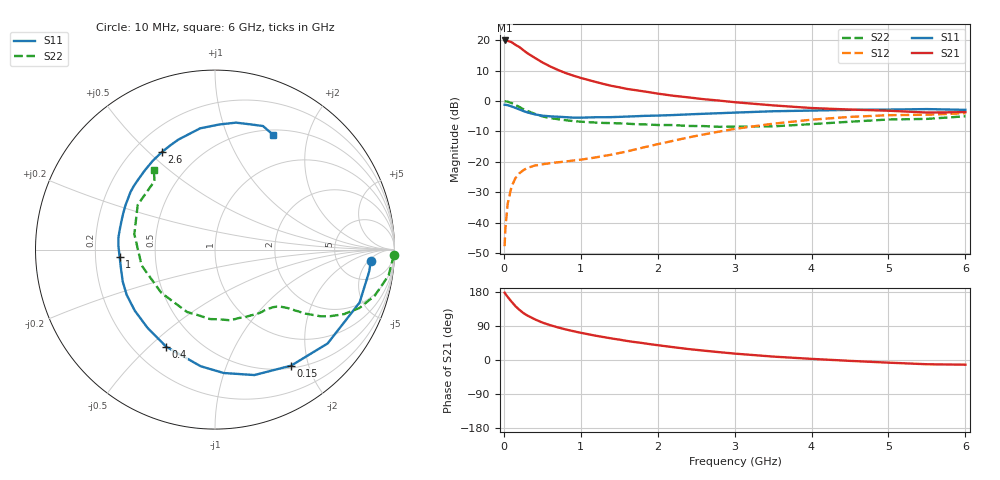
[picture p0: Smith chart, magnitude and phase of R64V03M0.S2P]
! SIEMENS Small Signal Semiconductors
! BFR193
! Si NPN RF Bipolar Junction Transistor in SOT23
! VCE = 4 V  IC = 3 mA
! Common Emitter S-Parameters:  May  1996
# GHz  S  MA  R  50
!  f  S11  S21  S12  S22
! GHz  MAG  ANG  MAG  ANG  MAG  ANG  MAG  ANG
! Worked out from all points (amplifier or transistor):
!   36 points, 10 MHz to 6 GHz, reference 50 ohm
!   highest |S21| = 20.0 dB at 10 MHz (marker M1)
!   |S21| within 3 dB of that: start of sweep to 244.1 MHz
!   unconditionally stable (mu >= 1): 1.043 GHz to 2.02 GHz
!   at 250 MHz: K = 0.31, MSG = 19.8 dB, |S12| = -22.8 dB
!   at 1.4 GHz: K = 1.10, MAG = 9.4 dB, |S12| = -17.6 dB
!   at 6 GHz: K = 0.98, MSG = 0.2 dB, |S12| = -4.0 dB
!   S11 on the Smith chart (normalised r, x): 10 MHz: 11, -6; 150 MHz: 0.54, -1.73; 400 MHz: 0.33, -0.57; 1 GHz: 0.31, -0.03; 2.6 GHz: 0.31, +0.55; 6 GHz: 0.56, +1.47
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0.01  0.8696 -4.2  9.946 177.6  0.0041 87.6  0.9953 -1.7
0.02  0.8681 -7.9  9.763 174.5  0.0081 83.7  0.9914 -3.3
0.05  0.858 -20.1  9.777 166.5  0.0205 79.3  0.9781 -8.4
0.1  0.8169 -39.8  9.339 153.9  0.0391 69.2  0.927 -16.0
0.15  0.7733 -56.7  8.433 142.2  0.0538 61.4  0.8684 -22.0
0.2  0.7325 -72.6  7.772 132.7  0.0644 55.3  0.8032 -26.6
0.25  0.6892 -86.0  6.948 124.5  0.0724 50.1  0.7403 -30.1
0.3  0.6547 -97.0  6.21 118.0  0.0789 46.8  0.6949 -32.3
0.4  0.6055 -116.7  5.174 107.6  0.0868 42.1  0.6175 -35.3
0.5  0.5754 -130.9  4.336 98.9  0.0911 40.1  0.5606 -37.2
0.6  0.5617 -142.7  3.728 92.1  0.0952 39.7  0.5256 -38.5
0.8  0.5441 -160.9  2.903 80.9  0.1013 41.1  0.485 -41.0
1  0.5329 -175.8  2.407 71.8  0.1087 45.3  0.4582 -44.3
1.1  0.5383 178.1  2.222 67.8  0.1134 47.6  0.4497 -46.4
1.3  0.5424 167.6  1.907 60.4  0.1252 51.9  0.4368 -50.6
1.6  0.5563 153.9  1.586 50.3  0.1484 57.1  0.4249 -58.3
2.2  0.589 131.9  1.225 33.9  0.2217 60.7  0.4033 -77.7
2.6  0.6186 118.6  1.074 24.7  0.2826 58.0  0.3879 -94.2
3.5  0.6806 97.0  0.85 9.0  0.4244 44.4  0.3841 -141.1
4.5  0.7169 80.6  0.726 -2.3  0.5494 25.3  0.4575 169.2
5.5  0.7385 68.8  0.648 -11.2  0.5963 6.8  0.5094 131.4
6  0.7174 63.3  0.658 -12.4  0.6313 1.5  0.5617 127.4
